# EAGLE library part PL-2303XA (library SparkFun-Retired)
Prolific USB chip, requires 12MHz xtal Never stocked
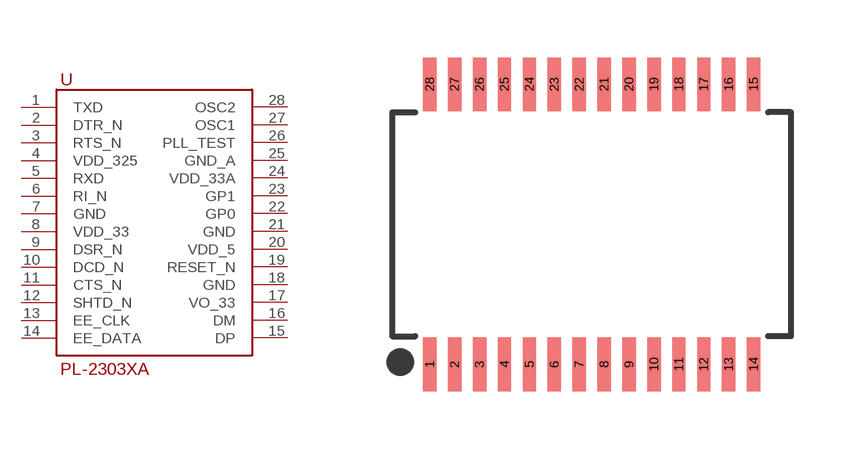
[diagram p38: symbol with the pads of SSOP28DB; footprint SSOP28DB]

Designator prefix -

## PL-2303XA  [SSOP28DB]
1  TXD
2  DTR_N
3  RTS_N
4  VDD_325
5  RXD
6  RI_N
7  GND
8  VDD_33
9  DSR_N
10  DCD_N
11  CTS_N
12  SHTD_N
13  EE_CLK
14  EE_DATA
15  DP
16  DM
17  VO_33
18  GND
19  RESET_N
20  VDD_5
21  GND
22  GP0
23  GP1
24  VDD_33A
25  GND_A
26  PLL_TEST
27  OSC1
28  OSC2

## Footprint SSOP28DB (pad centres in mm)
Small Shrink Outline Package
smd 0.348 x 1.397: 1 -4.225,-3.656; 2 -3.575,-3.656; 3 -2.925,-3.656; 4 -2.275,-3.656; 5 -1.625,-3.656; 6 -0.975,-3.656; 7 -0.325,-3.656; 8 0.325,-3.656; 9 0.975,-3.656; 10 1.625,-3.656; 11 2.275,-3.656; 12 2.925,-3.656; 13 3.575,-3.656; 14 4.225,-3.656; 15 4.225,3.656; 16 3.575,3.656; 17 2.925,3.656; 18 2.275,3.656; 19 1.625,3.656; 20 0.975,3.656; 21 0.325,3.656; 22 -0.325,3.656; 23 -0.975,3.656; 24 -1.625,3.656; 25 -2.275,3.656; 26 -2.925,3.656; 27 -3.575,3.656; 28 -4.225,3.656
